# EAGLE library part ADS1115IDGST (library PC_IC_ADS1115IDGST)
Analog-to-Digital Converter with Internal Reference
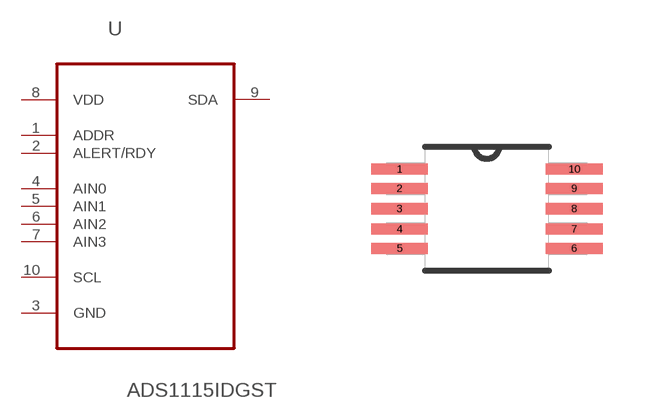
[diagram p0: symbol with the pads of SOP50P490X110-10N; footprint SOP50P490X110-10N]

Designator prefix U

## ADS1115IDGST (Availability: Unavailable; Description: 16-Bit ADC with Integrated MUX, PGA, Comparator, Oscillator, and Reference 10-VSSOP -40 to 125; MF: Texas Instruments; MP: ADS1115IDGST; Package: MSOP-10 Texas Instruments; Price: None)  [SOP50P490X110-10N]
1  ADDR  in
2  ALERT/RDY  in
3  GND  pas
4  AIN0  in
5  AIN1  in
6  AIN2  in
7  AIN3  in
8  VDD  pwr
9  SDA
10  SCL  in

## Footprint SOP50P490X110-10N (pad centres in mm)
smd 1.422 x 0.279: 1 -2.184,0.991; 2 -2.184,0.508; 3 -2.184,0; 4 -2.184,-0.508; 5 -2.184,-0.991; 6 2.184,-0.991; 7 2.184,-0.508; 8 2.184,0; 9 2.184,0.508; 10 2.184,0.991

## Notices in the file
This work is licensed under a Creative Commons Attribution-ShareAlike 4.0 International License (CC BY-SA) with Design Exception 1.0
